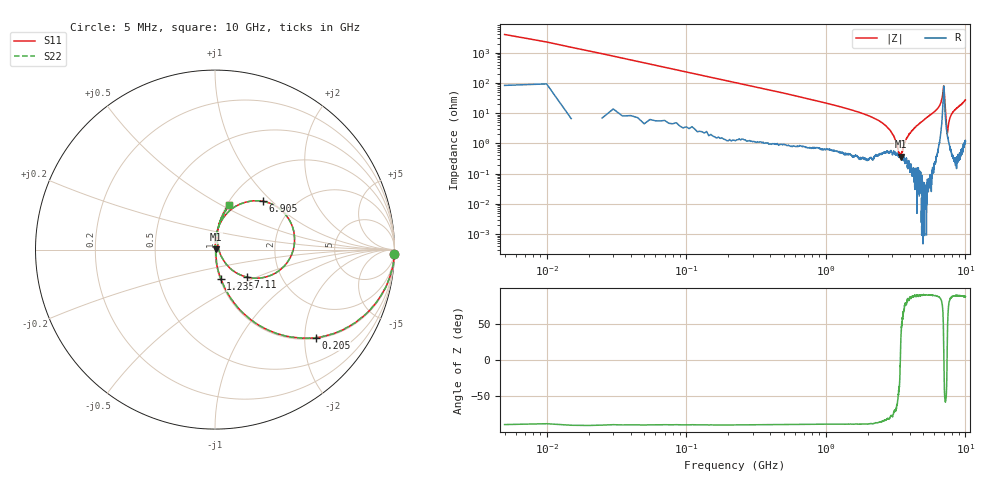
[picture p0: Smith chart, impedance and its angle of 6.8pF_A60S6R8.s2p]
! Amotech Co.,Ltd.
! http://www.amotech.co.kr/
! Part Number: A60S6R8
! These Parameters are Measured in Series Mode Connection
! Operation Temp=25[degC], DC Bias Voltage=0[V]
! Freq. Start=5[MHz] Stop=10[GHz], 2000[Steps]
! Date: Monday, July 13, 2020, 01:56:56
# GHZ S RI R 50.000000
!Freq.(Hz) S11(Real) S11(Imag) S21(Real) S21(Imag) S12(Real) S12(Imag) S22(Real) S22(Imag)
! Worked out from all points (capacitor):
!   2000 points, 5 MHz to 10 GHz, reference 50 ohm
!   read as one part in series: C = 6.89 pF near 55 MHz
!   lowest |Z| = 363 mohm at 3.445 GHz (marker M1)
!   series resonance near 3.421 GHz, so ESL is about 310 pH
!   S11 on the Smith chart (normalised r, x): 5 MHz: 3, -80; 205 MHz: 1.03, -2.26; 1.235 GHz: 1.01, -0.34; 6.905 GHz: 1.41, +0.89; 7.11 GHz: 1.36, -0.44; 10 GHz: 1.02, +0.55
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0.005  0.9989 -0.0251  0.00115 0.0251  0.00115 0.0251  0.9989 -0.0251
0.085  0.8761 -0.3207  0.1239 0.3207  0.1239 0.3207  0.8761 -0.3207
0.205  0.561 -0.4904  0.439 0.4904  0.439 0.4904  0.561 -0.4904
0.53  0.1612 -0.3579  0.8388 0.3579  0.8388 0.3579  0.1612 -0.3579
1.235  0.032 -0.1616  0.968 0.1616  0.968 0.1616  0.032 -0.1616
1.675  0.0161 -0.1096  0.9839 0.1096  0.9839 0.1096  0.0161 -0.1096
2.855  0.0058 -0.0281  0.9942 0.0281  0.9942 0.0281  0.0058 -0.0281
3.205  0.00422 -0.00968  0.9958 0.00968  0.9958 0.00968  0.00422 -0.00968
3.34  0.00386 -0.00301  0.9961 0.00301  0.9961 0.00301  0.00386 -0.00301
3.445  0.00326 0.00158  0.9967 -0.00158  0.9967 -0.00158  0.00326 0.00158
3.645  0.00362 0.00925  0.9964 -0.00925  0.9964 -0.00925  0.00362 0.00925
3.94  0.00272 0.0194  0.9973 -0.0194  0.9973 -0.0194  0.00272 0.0194
5.005  0.00297 0.0582  0.997 -0.0582  0.997 -0.0582  0.00297 0.0582
6.67  0.0652 0.2001  0.9348 -0.2001  0.9348 -0.2001  0.0652 0.2001
6.905  0.2678 0.2694  0.7322 -0.2694  0.7322 -0.2694  0.2678 0.2694
7  0.443 0.0404  0.557 -0.0404  0.557 -0.0404  0.443 0.0404
7.11  0.1808 -0.1539  0.8192 0.1539  0.8192 0.1539  0.1808 -0.1539
7.355  0.0248 -0.0127  0.9752 0.0127  0.9752 0.0127  0.0248 -0.0127
7.41  0.0194 0.00497  0.9806 -0.00497  0.9806 -0.00497  0.0194 0.00497
7.755  0.012 0.068  0.988 -0.068  0.988 -0.068  0.012 0.068
8.335  0.0173 0.1199  0.9827 -0.1199  0.9827 -0.1199  0.0173 0.1199
10  0.0792 0.2499  0.9208 -0.2499  0.9208 -0.2499  0.0792 0.2499
